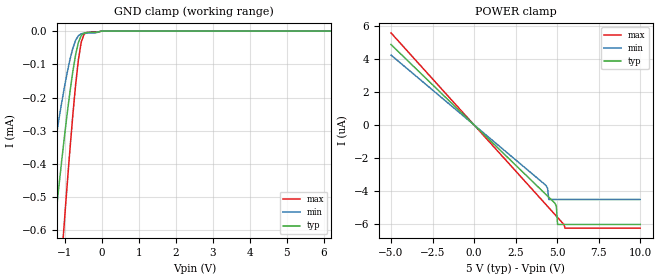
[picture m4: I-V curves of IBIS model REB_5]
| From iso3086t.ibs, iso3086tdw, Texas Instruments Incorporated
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|   REB_5 Model
[Model]   REB_5
Model_type   Input
Vinl   = 1.5V
Vinh   = 3.5V
|   typ   min   max
|   (nom PVT)   (Slow PVT)   (Fast PVT)
C_comp   0.25330759pF  0.25330759pF  0.25330760pF
[Model Spec]
Vinl   1.5V   1.35V   1.65V
Vinh   3.5V   3.15V   3.85V
[Voltage Range]   5   4.5   5.5
[Temperature Range]   40   125   -40
[Power Clamp Reference]   5   4.5   5.5
[GND Clamp Reference]   0   0   0
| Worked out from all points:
|   GND clamp passes 1 mA (typ) near -1.63 V on its own axis
[GND Clamp]
|   Voltage   I(typ)   I(min)   I(max)
-5V       -5.375mA   -3.708mA   -7.789mA
-1.608V   -969.8uA   -603.5uA   -1.558mA
-1.307V   -629.3uA   -373.6uA   -1.05mA
-1.231V   -548.1uA   -319.5uA   -926.8uA
-1.08V    -392uA     -216.7uA   -687.5uA
-1.005V   -318.1uA   -169uA     -572.1uA
-854.3mV  -181.8uA   -85.14uA   -353.7uA
-703.5mV  -71.78uA   -27.95uA   -162.8uA
-552.8mV  -13.69uA   -8.222uA   -34.02uA
-402mV    -4.439uA   -5.797uA   -4.04uA
0V        0A         0A         0A
10V       0A         0A         0A
[POWER Clamp]
|   Voltage   I(typ)   I(min)   I(max)
-5V       4.865uA    4.228uA    5.57uA
4.271V    -4.156uA   -3.612uA   -4.758uA
4.422V    -4.302uA   -3.827uA   -4.926uA
4.497V    -4.376uA   -4.51uA    -5.01uA
4.874V    -4.748uA   -4.51uA    -5.43uA
4.95V     -4.909uA   -4.51uA    -5.514uA
5.025V    -6.021uA   -4.51uA    -5.598uA
5.402V    -6.021uA   -4.51uA    -6.021uA
5.477V    -6.021uA   -4.51uA    -6.246uA
10V       -6.021uA   -4.51uA    -6.246uA
